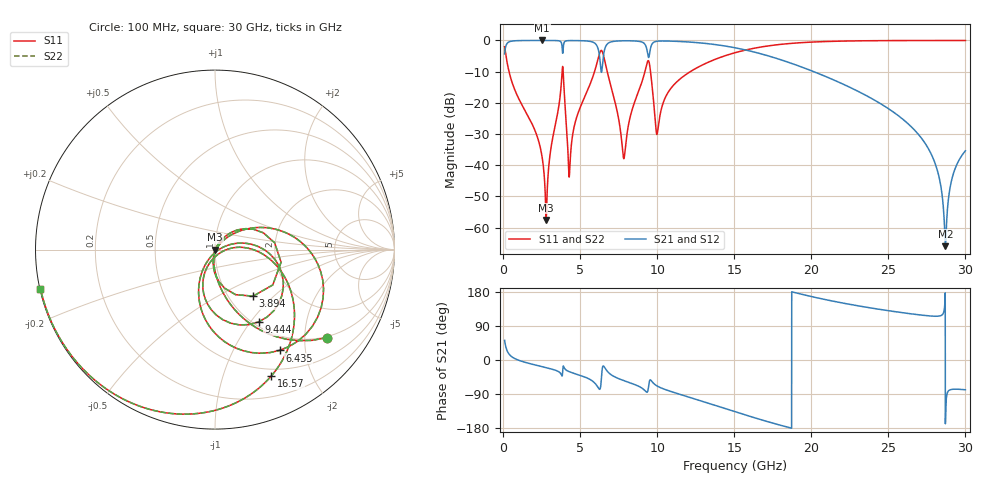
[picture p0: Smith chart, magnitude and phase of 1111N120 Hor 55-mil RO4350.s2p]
# GHz S MA R 50
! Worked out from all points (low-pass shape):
!   3201 points, 100 MHz to 30 GHz, reference 50 ohm
!   highest |S21| = -0.01 dB at 2.529 GHz (marker M1); lowest = -65.9 dB at 28.7 GHz (marker M2)
!   |S21| within 3 dB of the highest: 130.5 MHz to 3.845 GHz (3.714 GHz wide, 187 % of centre); 9.549 GHz to 15.69 GHz (6.142 GHz wide, 48.7 % of centre)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
!   lowest |S11| = -57.5 dB at 2.8 GHz (marker M3), VSWR 1.00, Z = 50.1 - j0.0357 ohm
!   |S11| at or under -10 dB: 387 MHz to 3.831 GHz (3.444 GHz wide, 163 % of centre); 6.759 GHz to 9.204 GHz (2.445 GHz wide, 30.6 % of centre); 9.569 GHz to 12.15 GHz (2.582 GHz wide, 23.8 % of centre)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
!   |S22| runs from -57.5 to 0.0 dB; largest |S21 - S12| = 0
!   S11 on the Smith chart (normalised r, x): 100 MHz: 0.97, -2.57; 3.894 GHz: 1.29, -0.75; 6.435 GHz: 0.77, -1.55; 9.444 GHz: 1.06, -1.10; 16.57 GHz: 0.42, -1.45; 30 GHz: 0.00, -0.11
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0.1  0.7935 -38.2  0.6083 51.8  0.6083 51.8  0.7935 -38.2
0.5671875  0.2189 -81.4  0.9752 8.5  0.9752 8.5  0.2189 -81.4
2.529375  0.01372 -102.8  0.9985 -17.5  0.9985 -17.5  0.01372 -102.8
2.800344  0.001326 -15.6  0.9984 -20.2  0.9984 -20.2  0.001326 -15.6
3.893562  0.335 -50.7  0.7027 -17.3  0.7027 -17.3  0.335 -50.7
4.304688  0.00689 -4.7  0.9933 -31.0  0.9933 -31.0  0.00689 -4.7
5.089563  0.09487 45.0  0.9894 -41.6  0.9894 -41.6  0.09487 45.0
6.023937  0.3757 16.5  0.8681 -64.3  0.8681 -64.3  0.3757 16.5
6.435062  0.6668 -57.4  0.3745 -23.3  0.3745 -23.3  0.6668 -57.4
6.771438  0.3068 -106.3  0.8805 -30.1  0.8805 -30.1  0.3068 -106.3
7.836625  0.01274 -51.9  0.9864 -54.4  0.9864 -54.4  0.01274 -51.9
9.44375  0.4703 -58.9  0.5328 -69.4  0.5328 -69.4  0.4703 -58.9
10.06978  0.04126 -16.4  0.974 -70.2  0.974 -70.2  0.04126 -16.4
11.27512  0.217 -0.4  0.9661 -88.1  0.9661 -88.1  0.217 -0.4
15.05  0.6352 -47.0  0.7626 -136.3  0.7626 -136.3  0.6352 -47.0
16.57303  0.7718 -66.1  0.6252 -155.5  0.6252 -155.5  0.7718 -66.1
20.03956  0.9407 -103.4  0.3246 167.2  0.3246 167.2  0.9407 -103.4
25.01978  0.9933 -140.7  0.08025 130.0  0.08025 130.0  0.9933 -140.7
27.74816  0.9966 -156.2  0.01574 116.1  0.01574 116.1  0.9966 -156.2
28.70122  0.9967 -161.0  0.000506 -168.2  0.000506 -168.2  0.9967 -161.0
29.18709  0.9967 -163.4  0.006877 -77.2  0.006877 -77.2  0.9967 -163.4
30  0.9966 -167.3  0.01705 -78.6  0.01705 -78.6  0.9966 -167.3
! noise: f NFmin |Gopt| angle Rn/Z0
0.1  0.0009264  0.8054  2.524  0.0009889
3.417  0.01488  0.6254  24.3  0.007123
6.743  0.104  0.8817  47.45  0.1599
10.06  0.06524  0.7484  68.18  0.03613
13.39  0.0444  0.5793  83.06  0.01135
16.7  0.06273  0.6475  97.91  0.01544
20.03  0.1041  0.7632  114.8  0.02708
23.35  0.2148  0.8784  133  0.0621
26.67  0.7573  0.9641  150.9  0.3049
30  1.632  0.9829  167.2  0.2785
